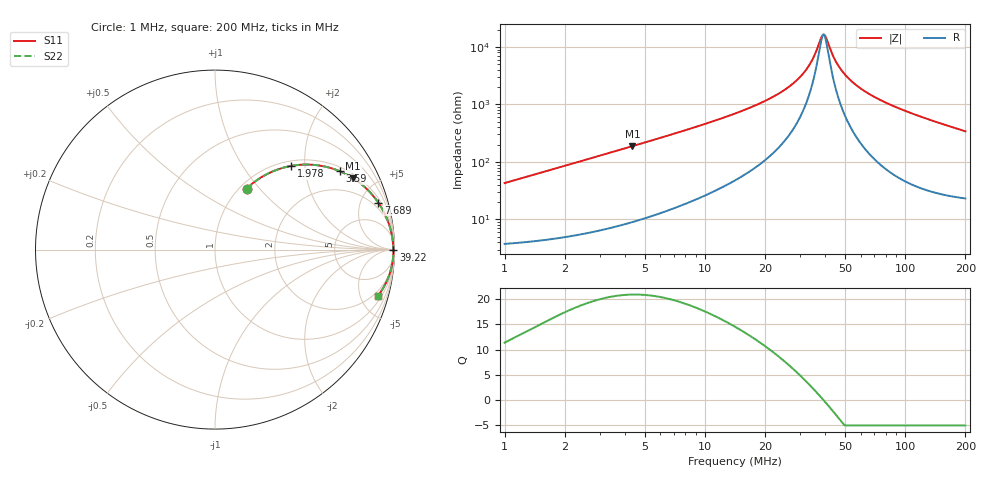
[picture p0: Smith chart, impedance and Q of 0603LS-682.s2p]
# MHz S MA R 50
!Freq  MagS11  AngS11  MagS21  AngS21  MagS12  AngS12  MagS22  AngS22
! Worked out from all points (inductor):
!   801 points, 1 MHz to 200 MHz, reference 50 ohm
!   read as one part in series: L = 6.8 uH near 1.027 MHz
!   highest Q = 20.9 at 4.35 MHz (marker M1), where L = 6.88 uH
!   self-resonance near 38.96 MHz
!   S11 on the Smith chart (normalised r, x): 1 MHz: 1.08, +0.85; 1.978 MHz: 1.10, +1.69; 3.59 MHz: 1.15, +3.09; 7.689 MHz: 1.35, +6.82; 39.22 MHz: open; 200 MHz: 1.46, -6.80
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1  0.3824 62.6  0.8911 -22.4  0.8911 -22.4  0.3824 62.6
1.978143  0.6292 47.8  0.7417 -38.9  0.7417 -38.9  0.6292 47.8
2.428972  0.7033 42.3  0.6745 -44.6  0.6745 -44.6  0.7033 42.3
3.59024  0.8219 32.0  0.5311 -55.2  0.5311 -55.2  0.8219 32.0
4.350466  0.8661 27.4  0.4601 -59.9  0.4601 -59.9  0.8661 27.4
5.86096  0.9165 20.9  0.3578 -66.3  0.3578 -66.3  0.9165 20.9
7.689473  0.9466 16.1  0.2771 -71.0  0.2771 -71.0  0.9466 16.1
14.14214  0.9803 8.1  0.1413 -78.0  0.1413 -78.0  0.9803 8.1
19.82466  0.9882 5.0  0.08709 -79.7  0.08709 -79.7  0.9882 5.0
25.3296  0.9915 3.1  0.05372 -79.3  0.05372 -79.3  0.9915 3.1
30.28922  0.9929 1.8  0.0315 -76.1  0.0315 -76.1  0.9929 1.8
34.35085  0.9936 0.9  0.01681 -67.1  0.01681 -67.1  0.9936 0.9
37.93865  0.9939 0.2  0.007162 -31.3  0.007162 -31.3  0.9939 0.2
39.216  0.994 -0.0  0.006051 1.8  0.006051 1.8  0.994 -0.0
40.26878  0.994 -0.2  0.00687 28.8  0.00687 28.8  0.994 -0.2
43.31193  0.994 -0.7  0.01338 63.1  0.01338 63.1  0.994 -0.7
45.36716  0.994 -1.0  0.01851 70.5  0.01851 70.5  0.994 -1.0
51.45067  0.9937 -1.9  0.03334 78.1  0.03334 78.1  0.9937 -1.9
62.75953  0.9924 -3.3  0.05834 80.9  0.05834 80.9  0.9924 -3.3
82.88649  0.9887 -5.6  0.09734 80.6  0.09734 80.6  0.9887 -5.6
123.3278  0.9768 -9.5  0.1654 77.2  0.1654 77.2  0.9768 -9.5
200  0.9424 -16.0  0.2764 70.1  0.2764 70.1  0.9424 -16.0
